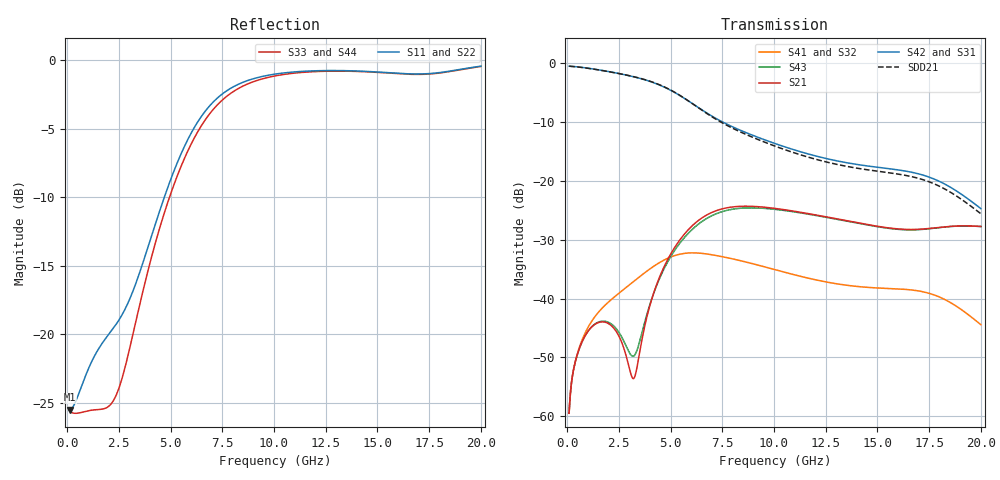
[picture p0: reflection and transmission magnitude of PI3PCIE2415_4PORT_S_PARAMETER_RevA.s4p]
! NPort=4 DATA=800 NOISE=0 GROUPDELAY=0 COMPLEX_DATAFORMAT=POLAR
! NumOfBlock=1 NumOfParam=0
! .MODEL Smodel S TSTONEFILE=PI3PCIE2415_4PORT_S_PARAMETER_RevA.s4p TYPE=S
!  -- The above .MODEL line can be used for the S element in the netlist.
! PORT DEFINITION
! PORT1 = INPUT+
! PORT2 = INPUT-
! PORT3 = OUTPUT+
! PORT4 = OUTPUT-
# Hz S MA R  50
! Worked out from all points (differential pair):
!   800 points, 100 MHz to 20 GHz, reference 50 ohm
!   strongest paths, dB at 100 MHz, 5.081 GHz, 10.06 GHz, 15.04 GHz, 20 GHz:
!     S42: -0.6, -4.8, -13.7, -17.7, -24.7
!     S31: -0.6, -4.8, -13.7, -17.7, -24.7
!     S21: -59.5, -32.0, -24.7, -27.8, -27.8
!     S43: -59.5, -32.5, -24.9, -27.8, -27.8
!     S41: -59.5, -32.9, -35.1, -38.2, -44.4
!     S32: -59.5, -32.9, -35.1, -38.2, -44.4
!   taken as a pair (ports 2,1 in; 4,3 out), SDD21 dB: -0.6, -4.8, -14.2, -18.4, -25.6
!   lowest |S11| = -25.5 dB at 124.9 MHz (marker M1), VSWR 1.11, Z = 55.3 - j1.82 ohm
!   |S11| at or under -10 dB: start of sweep to 4.703 GHz
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1e8  0.05305 -14.9  0.001064 75.3  0.9373 -2.8  0.001061 75.2
     0.001064 75.3  0.05305 -14.9  0.001061 75.2  0.9373 -2.8
     0.9373 -2.8  0.001061 75.2  0.05277 -12.2  0.001064 75.4
     0.001061 75.2  0.9373 -2.8  0.001064 75.4  0.05277 -12.2
1.24906e8  0.05296 -18.0  0.001285 72.5  0.9367 -3.5  0.001282 72.3
           0.001285 72.5  0.05296 -18.0  0.001282 72.3  0.9367 -3.5
           0.9367 -3.5  0.001282 72.3  0.05247 -14.7  0.001285 72.6
           0.001282 72.3  0.9367 -3.5  0.001285 72.6  0.05247 -14.7
1.44493e9  0.08637 -133.1  0.006176 41.6  0.8771 -37.2  0.007382 41.3
           0.006176 41.6  0.08637 -133.1  0.007382 41.3  0.8771 -37.2
           0.8771 -37.2  0.007382 41.3  0.05302 -126.9  0.006221 44.0
           0.007382 41.3  0.8771 -37.2  0.006221 44.0  0.05302 -126.9
3.06383e9  0.1363 125.4  0.002354 53.3  0.7738 -75.9  0.01328 15.8
           0.002354 53.3  0.1363 125.4  0.01328 15.8  0.7738 -75.9
           0.7738 -75.9  0.01328 15.8  0.09121 102.3  0.003357 60.1
           0.01328 15.8  0.7738 -75.9  0.003357 60.1  0.09121 102.3
7.04881e9  0.7013 -30.0  0.05424 67.5  0.3491 -159.9  0.02343 -83.2
           0.05424 67.5  0.7013 -30.0  0.02343 -83.2  0.3491 -159.9
           0.3492 -159.9  0.02343 -83.2  0.6587 -32.6  0.05095 66.5
           0.02343 -83.2  0.3492 -159.9  0.05095 66.5  0.6587 -32.6
1.04111e10  0.8967 -85.8  0.05705 10.2  0.1966 162.4  0.01689 -147.2
            0.05705 10.2  0.8967 -85.8  0.01689 -147.2  0.1966 162.4
            0.1966 162.4  0.01689 -147.1  0.8851 -86.1  0.05614 10.6
            0.01689 -147.1  0.1966 162.4  0.05614 10.6  0.8851 -86.1
2e10  0.9504 -128.8  0.04084 -32.3  0.05789 17.9  0.005989 39.4
      0.04084 -32.3  0.9504 -128.8  0.005989 39.4  0.05789 17.9
      0.05792 17.9  0.005992 39.5  0.9482 -128.8  0.04082 -32.0
      0.005992 39.5  0.05792 17.9  0.04082 -32.0  0.9482 -128.8
